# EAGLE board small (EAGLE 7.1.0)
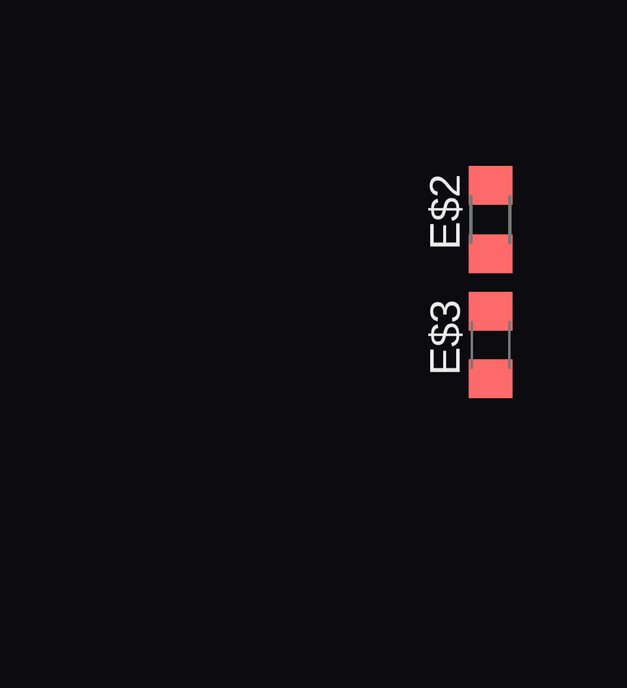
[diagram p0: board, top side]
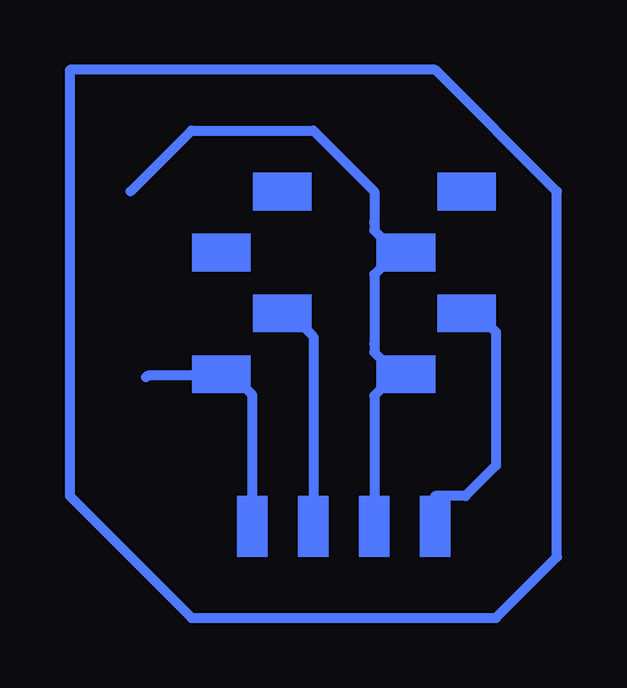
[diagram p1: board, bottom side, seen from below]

No outline drawn. Coordinates in mm, seen from the top.
Copper layers (1*16): Top 0.035mm / dielectric 1.5mm / Bottom 0.035mm
Design rules "default": minimum track width 10mil, minimum drill 24mil, track to track 8mil, track to pad 8mil, pad to pad 8mil, via to via 8mil, smd to smd 8mil, copper to edge 40mil, drill to drill 8mil, minimum pad ring 10mil, minimum via ring 8mil, stop-mask expansion 4mil, vias tented up to drill 0mil, thermal gap 10mil

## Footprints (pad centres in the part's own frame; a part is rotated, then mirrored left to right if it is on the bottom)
R1206 = smd 1.6 x 1.803: 1 -1.422,0; 2 1.422,0
C1206 = smd 1.6 x 1.8: 1 -1.4,0; 2 1.4,0

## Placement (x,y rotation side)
E$2  [R1206]  62,43.28 90 top
E$3  [C1206]  62,38.05 90 top

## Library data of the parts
E$2 E$3 = fab

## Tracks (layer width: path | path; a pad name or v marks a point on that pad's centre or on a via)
S$1
  Bottom 0.406: 57.15,31.17 57.15,35.97 58.06,36.88
S$2
  Bottom 0.406: 52.07,30.48 52.07,35.94 51.36,36.65
S$3
  Bottom 0.406: 49.53,31.75 48.26,31.75 46.99,33.02 46.99,38.58 47.85,39.45
S$4
  Bottom 0.406: 54.61,30.48 54.61,38.41 55.37,39.17
S$5
  Bottom 0.406: 49.53,49.53 64.77,49.53 64.77,31.75 59.69,26.67 46.99,26.67 44.45,29.21 44.45,44.45 49.53,49.53
S$6
  Bottom 0.406: 62.23,44.45 59.69,46.99 54.61,46.99 52.07,44.45 52.07,43.18
S$7
  Bottom 0.406: 52.07,38.1 52.07,41 51.56,41.5
S$8
  Bottom 0.406: 52.07,43.13 52.07,42.82 51.38,42.14
S$9
  Bottom 0.406: 52.07,38.08 52.07,37.74 51.56,37.24
S$10
  Bottom 0.406: 58.95,36.78 61.52,36.78 61.59,36.7
(copper drawn outside any net)
  shapes: Bottom area x12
